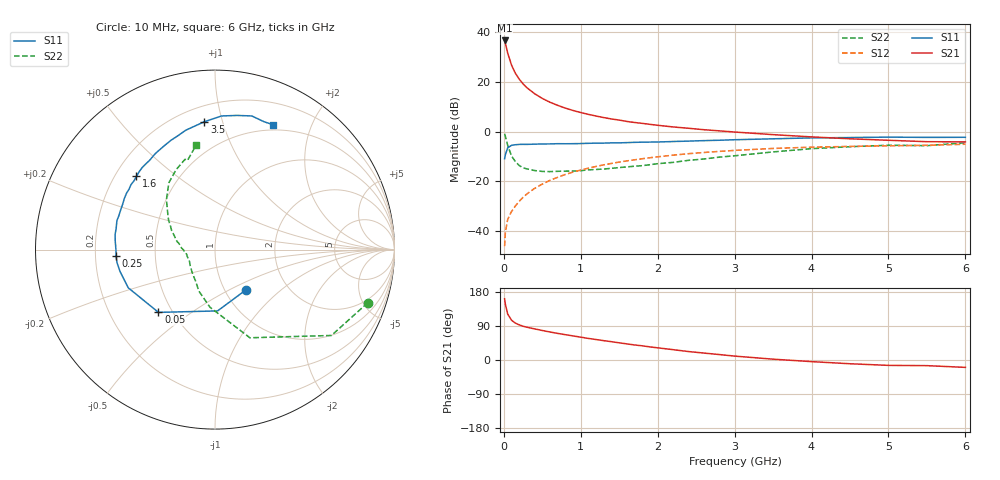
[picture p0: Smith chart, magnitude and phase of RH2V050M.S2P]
! SIEMENS Small Signal Semiconductors
! BFR106
! Si NPN RF Bipolar Junction Transistor in SOT23
! VCE = 2 V  IC = 50 mA
! Common Emitter S-Parameters:  August  1996
# GHz  S  MA  R  50
!  f  S11  S21  S12  S22
! GHz  MAG  ANG  MAG  ANG  MAG  ANG  MAG  ANG
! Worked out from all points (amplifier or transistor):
!   36 points, 10 MHz to 6 GHz, reference 50 ohm
!   highest |S21| = 36.7 dB at 10 MHz (marker M1)
!   |S21| within 3 dB of that: start of sweep to 34.27 MHz
!   unconditionally stable (mu >= 1): 227.3 MHz to 2.747 GHz; 5.149 GHz to end of sweep
!   at 250 MHz: K = 1.02, MAG = 22.0 dB, |S12| = -26.5 dB
!   at 1.4 GHz: K = 1.06, MAG = 7.4 dB, |S12| = -12.8 dB
!   at 6 GHz: K = 1.01, MAG = -0.1 dB, |S12| = -5.1 dB
!   S11 on the Smith chart (normalised r, x): 10 MHz: 1.24, -0.61; 50 MHz: 0.42, -0.38; 250 MHz: 0.29, -0.03; 1.6 GHz: 0.29, +0.37; 3.5 GHz: 0.30, +0.87; 6 GHz: 0.44, +1.47
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0.01  0.2831 -53.1  68.59 161.5  0.0049 78.3  0.9011 -19.2
0.02  0.3419 -87.6  60.29 147.0  0.0094 67.4  0.8061 -36.4
0.05  0.4707 -132.0  38.26 121.3  0.0169 59.5  0.5284 -68.4
0.1  0.528 -156.2  21.85 105.0  0.0245 60.3  0.3223 -95.0
0.15  0.5428 -166.9  14.96 97.3  0.0317 63.6  0.2481 -111.2
0.2  0.5503 -172.1  11.4 92.7  0.0393 66.7  0.2069 -121.4
0.25  0.5527 -176.2  9.124 89.1  0.0473 68.6  0.1861 -131.2
0.3  0.5514 -179.3  7.649 86.5  0.0553 69.7  0.1767 -137.2
0.4  0.5579 175.1  5.791 82.1  0.0716 70.7  0.1639 -147.5
0.5  0.5628 171.2  4.652 77.9  0.0874 70.7  0.1571 -154.5
0.6  0.5637 167.5  3.9 73.9  0.1039 70.1  0.156 -158.9
0.7  0.5698 163.6  3.372 70.2  0.12 69.0  0.1581 -162.9
0.9  0.5699 157.4  2.659 63.5  0.1523 66.4  0.1596 -170.4
1.1  0.5796 150.7  2.218 56.9  0.1833 63.4  0.1691 -174.6
1.3  0.5854 144.9  1.913 51.0  0.2137 60.2  0.1758 -179.6
1.6  0.599 136.9  1.599 42.5  0.2564 55.3  0.194 174.2
2.2  0.6301 121.8  1.239 27.3  0.3347 45.2  0.2394 161.2
2.8  0.6683 107.7  1.034 14.4  0.3984 35.2  0.3052 147.8
3.5  0.7148 94.8  0.867 2.2  0.4569 24.3  0.3889 134.1
4.5  0.7577 80.6  0.715 -9.9  0.502 10.0  0.4948 116.0
5.5  0.763 69.0  0.625 -14.9  0.5287 1.4  0.5202 107.1
6  0.7668 65.3  0.62 -19.5  0.5555 -5.4  0.5944 100.0
